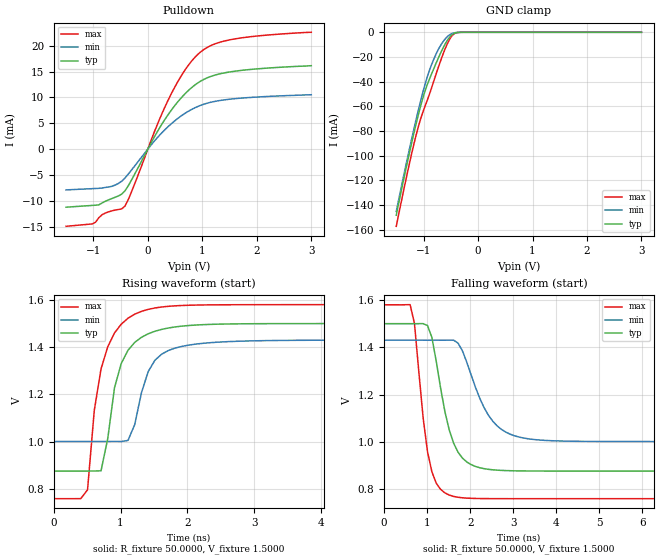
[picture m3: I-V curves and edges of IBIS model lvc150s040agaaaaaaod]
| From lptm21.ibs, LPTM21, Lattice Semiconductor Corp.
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|   Model lvc150s040agaaaaaaod
[Model]   lvc150s040agaaaaaaod
Model_type   I/O_open_drain
Polarity   Non-Inverting
Enable   Active-Low
Vinl =   0.3750V
Vinh =   1.1250V
Vmeas =   0.7500V
Cref =   0.0F
Rref =   1.0000M
Vref =   0.0V
C_comp   4.2000pF   3.8000pF   7.5000pF
[Temperature Range]   25.0000   0.1050k   -40.0000
[Voltage Range]   1.5000V   1.4300V   1.5800V
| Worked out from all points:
|   slope of the pulldown table from 0 to 0.225 V, typ, clamps not added: 52.9 ohm
|   GND clamp passes 1 mA (typ) near -0.44 V on its own axis
|   rising waveform, R_fixture 50.0000, V_fixture 1.5000: 20-80 % time 291ps typ, 291ps min, 289ps max; typ from 0.876 V to 1.5 V
|   falling waveform, R_fixture 50.0000, V_fixture 1.5000: 20-80 % time 426ps typ, 620ps min, 302ps max; typ from 1.5 V to 0.876 V
[Pulldown]
|Voltage   I(typ)   I(min)   I(max)
-1.5V     -11.23mA   -7.89mA    -14.93mA
-1.02V    -10.89mA   -7.649mA   -14.47mA
-900mV    -10.78mA   -7.588mA   -13.29mA
-600mV    -9.318mA   -6.96mA    -11.79mA
-420mV    -8.084mA   -5.596mA   -11.02mA
180mV     3.467mA    2.274mA    4.899mA
360mV     6.469mA    4.221mA    9.187mA
660mV     10.45mA    6.76mA     14.94mA
960mV     13.08mA    8.424mA    18.71mA
1.2V      14.21mA    9.162mA    20.22mA
1.56V     15.01mA    9.71mA     21.24mA
3V        16.13mA    10.51mA    22.59mA
[GND_clamp]
|Voltage   I(typ)   I(min)   I(max)
-1.5V     -148.1mA   -145.1mA   -157.1mA
-1.32V    -110mA     -107mA     -118.7mA
-1.17V    -80.46mA   -77.1mA    -89.31mA
-1.05V    -59.23mA   -55mA      -69.72mA
-930mV    -42.26mA   -35.91mA   -54.92mA
-810mV    -29.29mA   -21.6mA    -39.3mA
-690mV    -17.13mA   -10.88mA   -23.54mA
-600mV    -9.258mA   -5.26mA    -13.05mA
-540mV    -5.061mA   -2.654mA   -7.228mA
-450mV    -1.178mA   -585.4uA   -1.585mA
-300mV    -18.71uA   -15.93uA   -16.54uA
3V        0A         0A         0A
[Ramp]
| variable   typ   min   max
dV/dt_r  0.3746/0.2882n   0.2575/0.2879n   0.4927/0.2859n
dV/dt_f  0.3746/0.4213n   0.2575/0.6133n   0.4927/0.2991n
R_load = 50.0000
[Rising Waveform]
R_fixture=   50.0000
V_fixture=   1.5000
V_fixture_min=   1.4300
V_fixture_max=   1.5800
|time   V(typ)   V(min)   V(max)
0s        875.7mV    1.001V     758.8mV
505.1ps   875.7mV    1.001V     796.4mV
606.1ps   876mV      1.001V     1.133V
707.1ps   876.9mV    1.001V     1.308V
1.01ns    1.331V     1.001V     1.498V
1.212ns   1.42V      1.073V     1.54V
1.414ns   1.457V     1.297V     1.56V
1.717ns   1.481V     1.386V     1.573V
2.525ns   1.498V     1.422V     1.579V
10ns      1.5V       1.43V      1.58V
[Falling Waveform]
R_fixture=   50.0000
V_fixture=   1.5000
V_fixture_min=   1.4300
V_fixture_max=   1.5800
|time   V(typ)   V(min)   V(max)
0s        1.5V       1.43V      1.58V
606.1ps   1.5V       1.43V      1.581V
707.1ps   1.5V       1.43V      1.501V
1.01ns    1.492V     1.43V      957.7mV
1.212ns   1.341V     1.43V      824.5mV
1.515ns   1.049V     1.43V      774mV
2.02ns    903.3mV    1.284V     760.3mV
2.525ns   881.1mV    1.087V     759mV
3.131ns   876.5mV    1.02V      758.8mV
10ns      875.7mV    1.001V     758.8mV
